TYPE STR_AI :
STRUCT
VG101_Pressure	,
VG102_Pressure	,
VG103_Pressure	,
VG104_Pressure	,
BA1_Pressure	,
MFC1_Flow	,
MFC2_Flow	,
MFC3_Flow	,
MFC4_Flow	,
MFC5_Flow	,
MFC6_Flow	,
MFC7_Flow	,
CHILLER1_TEMP_PV	,
CHILLER1_DI_PV	,
CHILLER1_FLOW_PV	,
CHILLER1_PRESS_PV	,
CHILLER2_TEMP_PV	,
CHILLER2_DI_PV	,
CHILLER2_FLOW_PV	,
CHILLER2_PRESS_PV	,
Turbo_Pump_Temp	,
APC_Temp	,	//TC01
Gate_Valve_Temp	,		//TC13
Gate_Valve_Temp_Monitor,	//TC14
IGS_Temp1	,	//TC35
IGS_Temp2	,	//TC36
IGS_Temp3	,	//TC35
IGS_Temp4	,	//TC36
Lid_Temp	,	//TC02
Lid_Temp_Monitor1	,	//TC03
Lid_Temp_Monitor2	,	//TC04
Tape_Temp1	,	//TC31
Tape_Temp2	,	//TC32
AV102_Temp	,
AV101_Temp	,
AV104_Temp	,
AV105_Temp	,
//BA01_Temp	,
//VG103_Pipe_Temp	,
Exhaust1_3_Temp	,
Exhaust4_7_Temp	,
VG101_Pipe_Temp	,
Chamber_Temp1	,	//TC05
Chamber_Temp2	,	//TC06
Chamber_Temp3	,	//TC07
Chamber_Temp_Monitor,	//TC12
Stage_Temp1	,		//TC08
Stage_Temp1_Monitor	,
Stage_Temp2	,		//TC09
Stage_Temp2_Monitor	,
Stage_Temp3	,		//TC10
Stage_Temp3_Monitor	,
Stage_Temp4	,
Stage_Temp4_Monitor	:REAL;		//TC11	

PG_PS1_Value	,
PG_PS2_Value	,
PG_PS3_Value	,
PG_PS4_Value	,
PG_PS5_Value	,
PG_PS6_Value	,
PG_PS7_Value	,
PG_PS8_Value	,
PG_PS9_Value	,
PS1_Value	,
PS2_Value	,
MS1_Value	,
GD01_Value	,
GD02_Value	:REAL;

APC:VAT_IN;

TMP:TMP_IN;

VG103_PV	,//原PG10

VG101_PV	,//原PS10

VG102_PV	,//原PS11

BA1_PV	,

VG104_PV:REAL;//原PS12

Water_Flow:REAL;

END_STRUCT
END_TYPE
